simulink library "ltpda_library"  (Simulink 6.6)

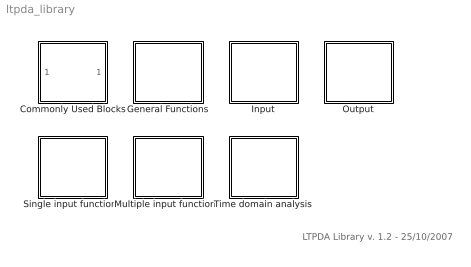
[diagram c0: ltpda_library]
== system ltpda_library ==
  note: LTPDA Library v. 1.2 - 25/10/2007
  Commonly Used Blocks : Subsystem
  General Functions : Subsystem
  Input : Subsystem
  Multiple input functions : Subsystem
  Output : Subsystem
  Single input functions : Subsystem
  Time domain analysis : Subsystem

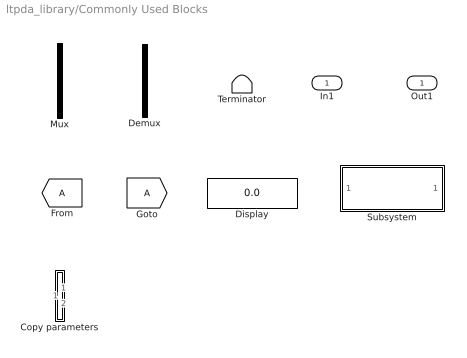
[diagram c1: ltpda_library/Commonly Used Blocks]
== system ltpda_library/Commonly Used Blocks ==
  In1 : Inport
  Copy parameters : Subsystem
  Demux : Demux  Outputs=2
  Display : Display
  Mux : Mux  Tag=mux  Inputs=2
  Subsystem : Subsystem
  Terminator : Terminator
  Out1 : Outport

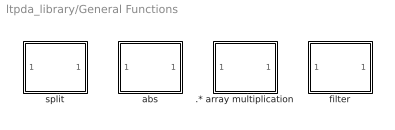
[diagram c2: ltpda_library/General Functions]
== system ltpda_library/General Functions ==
  .* array multiplication : Subsystem
  abs : Subsystem
  filter : Subsystem  Tag=freepl
  split : Subsystem  Tag=freepl

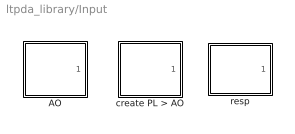
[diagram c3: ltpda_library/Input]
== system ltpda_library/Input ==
  AO : Subsystem  Tag=input
  create PL > AO : Subsystem  Tag=freepl
  resp : Subsystem  Tag=freepl

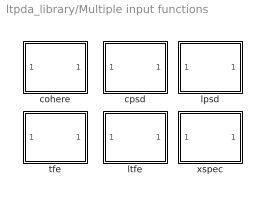
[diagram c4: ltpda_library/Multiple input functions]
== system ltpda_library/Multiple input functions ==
  cohere : Subsystem  Tag=function
  cpsd : Subsystem  Tag=function
  lpsd : Subsystem  Tag=function
  ltfe : Subsystem  Tag=function
  tfe : Subsystem  Tag=function
  xspec : Subsystem  Tag=function

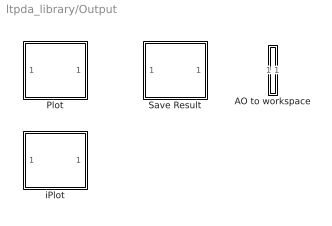
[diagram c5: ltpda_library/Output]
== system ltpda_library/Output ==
  AO to workspace : Subsystem
  Plot : Subsystem
  Save Result : Subsystem
  iPlot : Subsystem

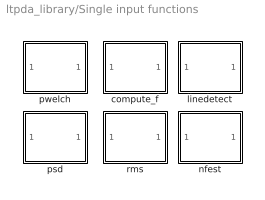
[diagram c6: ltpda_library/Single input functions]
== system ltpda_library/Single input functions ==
  compute_f : Subsystem  Tag=function
  linedetect : Subsystem  Tag=function
  nfest : Subsystem  Tag=function
  psd : Subsystem  Tag=function
  pwelch : Subsystem  Tag=function
  rms : Subsystem  Tag=function

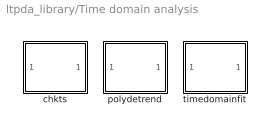
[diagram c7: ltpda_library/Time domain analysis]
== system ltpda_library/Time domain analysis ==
  chkts : Subsystem  Tag=function
  polydetrend : Subsystem  Tag=function
  timedomainfit : Subsystem  Tag=function

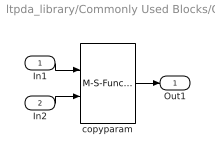
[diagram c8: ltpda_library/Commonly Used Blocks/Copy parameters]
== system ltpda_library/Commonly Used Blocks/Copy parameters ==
  In1 : Inport
  In2 : Inport  Port=2
  copyparam : M-S-Function  FunctionName=copyparam
  Out1 : Outport
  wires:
  copyparam/1 -> Out1/1
  In1/1 -> copyparam/1
  In2/1 -> copyparam/2

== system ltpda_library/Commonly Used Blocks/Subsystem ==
  In1 : Inport
  Out1 : Outport
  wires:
  In1/1 -> Out1/1

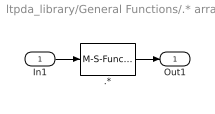
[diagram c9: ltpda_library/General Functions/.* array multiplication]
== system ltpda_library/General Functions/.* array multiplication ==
  In1 : Inport
  .* : M-S-Function  Tag=abs  FunctionName=ltpdaarrmult
  Out1 : Outport
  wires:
  .*/1 -> Out1/1
  In1/1 -> .*/1

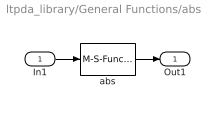
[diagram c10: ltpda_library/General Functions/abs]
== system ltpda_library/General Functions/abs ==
  In1 : Inport
  abs : M-S-Function  Tag=abs  FunctionName=ltpdasim
  Out1 : Outport
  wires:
  In1/1 -> abs/1
  abs/1 -> Out1/1

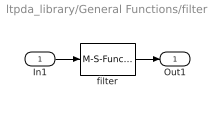
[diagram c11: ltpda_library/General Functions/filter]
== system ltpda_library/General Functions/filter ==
  In1 : Inport
  filter : M-S-Function  Tag=filter  FunctionName=ltpdasim
  Out1 : Outport
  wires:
  In1/1 -> filter/1
  filter/1 -> Out1/1

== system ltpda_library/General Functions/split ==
  In1 : Inport
  split : M-S-Function  Tag=split  FunctionName=ltpdasim
  Out1 : Outport
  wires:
  split/1 -> Out1/1
  In1/1 -> split/1

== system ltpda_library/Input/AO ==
  Input : Constant  Value=0
  Input AO : Outport
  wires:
  Input/1 -> Input AO/1

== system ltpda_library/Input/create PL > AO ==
  ltpdapl2ao : M-S-Function  FunctionName=ltpdapl2ao
  Out1 : Outport
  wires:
  ltpdapl2ao/1 -> Out1/1

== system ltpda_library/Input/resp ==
  resp : M-S-Function  Tag=resp  FunctionName=ltpdaresp
  Out1 : Outport
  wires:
  resp/1 -> Out1/1

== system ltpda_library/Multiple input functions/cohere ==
  In1 : Inport
  ltpda_cohere : M-S-Function  Tag=ltpda_cohere  FunctionName=ltpdasimmulti
  Out1 : Outport
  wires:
  ltpda_cohere/1 -> Out1/1
  In1/1 -> ltpda_cohere/1

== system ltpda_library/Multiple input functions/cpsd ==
  In1 : Inport
  ltpda_cpsd : M-S-Function  Tag=ltpda_cpsd  FunctionName=ltpdasimmulti
  Out1 : Outport
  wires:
  ltpda_cpsd/1 -> Out1/1
  In1/1 -> ltpda_cpsd/1

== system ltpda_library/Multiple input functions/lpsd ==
  In1 : Inport
  ltpda_lpsd : M-S-Function  Tag=ltpda_lpsd  FunctionName=ltpdasimmulti
  Out1 : Outport
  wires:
  In1/1 -> ltpda_lpsd/1
  ltpda_lpsd/1 -> Out1/1

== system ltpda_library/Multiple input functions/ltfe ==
  In1 : Inport
  ltpda_ltfe : M-S-Function  Tag=ltpda_ltfe  FunctionName=ltpdasimmulti
  Out1 : Outport
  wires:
  In1/1 -> ltpda_ltfe/1
  ltpda_ltfe/1 -> Out1/1

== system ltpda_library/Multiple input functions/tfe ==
  In1 : Inport
  ltpda_tfe : M-S-Function  Tag=ltpda_tfe  FunctionName=ltpdasimmulti
  Out1 : Outport
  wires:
  ltpda_tfe/1 -> Out1/1
  In1/1 -> ltpda_tfe/1

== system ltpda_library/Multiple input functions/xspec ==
  In1 : Inport
  ltpda_xspec : M-S-Function  Tag=ltpda_xspec  FunctionName=ltpdasimmulti
  Out1 : Outport
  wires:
  ltpda_xspec/1 -> Out1/1
  In1/1 -> ltpda_xspec/1

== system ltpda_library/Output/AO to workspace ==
  In1 : Inport
  aotoworkspace : M-S-Function  Tag=ltpda_pwelch  FunctionName=aotoworkspace
  Out1 : Outport
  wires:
  In1/1 -> aotoworkspace/1
  aotoworkspace/1 -> Out1/1

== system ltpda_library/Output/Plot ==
  In1 : Inport
  plot : M-S-Function  FunctionName=ltpdaplot
  Out1 : Outport
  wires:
  plot/1 -> Out1/1
  In1/1 -> plot/1

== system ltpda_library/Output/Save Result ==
  In1 : Inport
  save result : M-S-Function  FunctionName=saveresultao
  Out1 : Outport
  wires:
  In1/1 -> save result/1
  save result/1 -> Out1/1

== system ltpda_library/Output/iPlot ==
  In1 : Inport
  iplot : M-S-Function  FunctionName=ltpdaiplot
  Out1 : Outport
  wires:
  In1/1 -> iplot/1
  iplot/1 -> Out1/1

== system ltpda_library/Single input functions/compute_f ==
  In1 : Inport
  ltpda_compute_f : M-S-Function  Tag=ltpda_compute_f  FunctionName=ltpdasim
  Out1 : Outport
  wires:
  ltpda_compute_f/1 -> Out1/1
  In1/1 -> ltpda_compute_f/1

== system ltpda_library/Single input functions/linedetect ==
  In1 : Inport
  ltpda_linedetect : M-S-Function  Tag=ltpda_linedetect  FunctionName=ltpdasim
  Out1 : Outport
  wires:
  In1/1 -> ltpda_linedetect/1
  ltpda_linedetect/1 -> Out1/1

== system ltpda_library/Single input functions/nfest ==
  In1 : Inport
  ltpda_nfest : M-S-Function  Tag=ltpda_nfest  FunctionName=ltpdasim
  Out1 : Outport
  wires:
  ltpda_nfest/1 -> Out1/1
  In1/1 -> ltpda_nfest/1

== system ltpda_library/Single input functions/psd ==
  In1 : Inport
  ltpda_psd : M-S-Function  Tag=ltpda_psd  FunctionName=ltpdasim
  Out1 : Outport
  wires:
  ltpda_psd/1 -> Out1/1
  In1/1 -> ltpda_psd/1

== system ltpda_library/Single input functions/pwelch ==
  In1 : Inport
  ltpda_pwelch : M-S-Function  Tag=ltpda_pwelch  FunctionName=ltpdasim
  Out1 : Outport
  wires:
  In1/1 -> ltpda_pwelch/1
  ltpda_pwelch/1 -> Out1/1

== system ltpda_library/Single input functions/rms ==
  In1 : Inport
  ltpda_rms : M-S-Function  Tag=ltpda_rms  FunctionName=ltpdasim
  Out1 : Outport
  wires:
  In1/1 -> ltpda_rms/1
  ltpda_rms/1 -> Out1/1

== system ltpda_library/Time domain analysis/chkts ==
  In1 : Inport
  ltpda_chkts : M-S-Function  Tag=ltpda_chkts  FunctionName=ltpdasim
  Out1 : Outport
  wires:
  ltpda_chkts/1 -> Out1/1
  In1/1 -> ltpda_chkts/1

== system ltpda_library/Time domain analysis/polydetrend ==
  In1 : Inport
  ltpda_polydetrend : M-S-Function  Tag=ltpda_polydetrend  FunctionName=ltpdasim
  Out1 : Outport
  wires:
  In1/1 -> ltpda_polydetrend/1
  ltpda_polydetrend/1 -> Out1/1

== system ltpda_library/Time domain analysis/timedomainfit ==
  In1 : Inport
  ltpda_timedomainfit : M-S-Function  Tag=ltpda_timedomainfit  FunctionName=ltpdasim
  Out1 : Outport
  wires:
  ltpda_timedomainfit/1 -> Out1/1
  In1/1 -> ltpda_timedomainfit/1
